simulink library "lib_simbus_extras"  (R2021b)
settings: Solver=ode45  StartTime=0.0  StopTime=10.0  RelTol=1e-3  EnableMultiTasking=on
undefined symbols (not defined in the file): BLOCKS, core, generic_inertance_pvs, measurement, SIMBUS, SIMBUS_BONDGRAPHS, SIMBUS_CORE, Timeseries
libraries: lib_select_power_variable x3

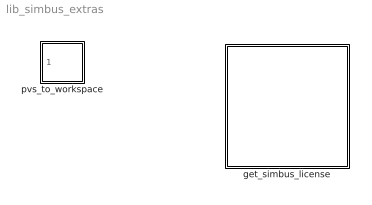
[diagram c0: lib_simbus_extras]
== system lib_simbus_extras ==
  get_simbus_license : Subsystem  mask(Get Simbus Products License){simbus_vendor=SIMBUS, simbus_toolbox=SIMBUS_CORE, simbus_component=BLOCKS, simbus_class=core.utils.get_simbus_license}
      mask prompts: simbus_vendor "Vendor:"; simbus_toolbox "Toolbox:"; simbus_component "Component:"; simbus_class "Class:"
      mask help: If you discover one or more missing library block in this model, then it is likely that you do not have a license to use Simbus products. Select the license that is most appropriate to your needs using one of the buttons below. If you are in receipt of this model from a third party (such as a project partner, contractor, or consultant) but do not need to modify it, then select the free Run-Time License. A Run-Time License is perpetual. If you wish to evaluate Simbus products for free, then select the free Trial License. A Trial License is a limited-duration license but is not limited in any wa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
  pvs_to_workspace : Subsystem  mask(Power Variables to Workspace){simbus_vendor=SIMBUS, simbus_toolbox=SIMBUS_BONDGRAPHS, simbus_component=BLOCKS, simbus_class=measurement.pvs_to_workspace, msk_var_name=generic_inertance_pvs, msk_max_datapoints=inf, msk_decimation=1, msk_save_format=Timeseries, msk_sample_time=-1, msk_apply_antialiasing=off}
      mask prompts: simbus_vendor "Vendor:"; simbus_toolbox "Toolbox:"; simbus_component "Component:"; simbus_class "Class:"; msk_var_name "Simulink:blkprm_prompts:ToWksVarName"; msk_max_datapoints "Simulink:blkprm_prompts:ToWksMaxDataPoints"; msk_decimation "Simulink:blkprm_prompts:AllBlksDecimation"; msk_save_format "Simulink:blkprm_prompts:ToWksSaveFormat"; msk_sample_time "Simulink:blkprm_prompts:AllBlksSampleTime"; msk_apply_antialiasing "Apply Antialiasing Filtering?"
      mask help: This block saves the generalized effort, generalized flow, and power of the connected bond to the MATLAB workspace. The user may optionally specify antialiasing filtering for these signals. The antialiasing filters are simple first-order filters with a cut-off frequency in Hertz set 1/(2*T), where T is a the sample period.
      mask init:
      | this_blk_bio = simbus_bio.factory(gcb);
      | apply_antialiasing = this_blk_bio{'apply_antialiasing'};
      | if apply_antialiasing
      | 
      |    Ts = this_blk_bio{'sample_time'};
      |    if Ts < 0
      |       errordlg('Failed to determine sample time.');
      |    elseif Ts > 0
      |       w_break = (pi/Ts);
      |       num_f = w_break;
      |       den_f = [1, w_break];
      |    else
      |       num_f = 1;
      |       den_f = 1;
      |    end % if Ts < 0
      | else % "apply_antialiasing" is false => pass-through
      | 
      |    num_f = 1;
      |    den_f = 1;
      | 
      | end % if apply_antialiasing

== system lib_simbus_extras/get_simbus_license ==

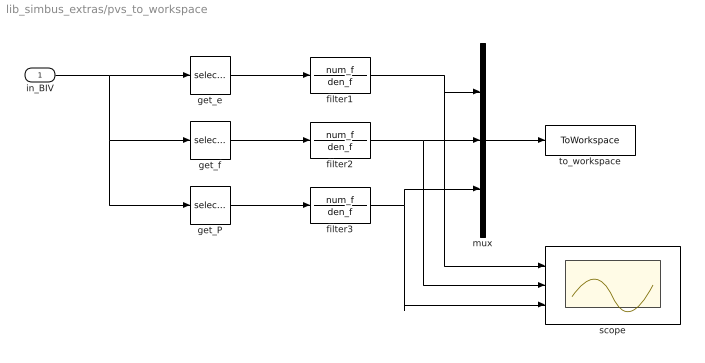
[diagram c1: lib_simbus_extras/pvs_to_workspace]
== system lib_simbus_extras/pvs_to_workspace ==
  in_BIV : Inport
  filter1 : TransferFcn  Numerator=num_f  Denominator=den_f
  filter2 : TransferFcn  Numerator=num_f  Denominator=den_f
  filter3 : TransferFcn  Numerator=num_f  Denominator=den_f
  get_P : lib_select_power_variable/select_power_variable  simbus_vendor=SIMBUS  simbus_toolbox=SIMBUS_BONDGRAPHS  simbus_component=BLOCKS  simbus_class=measurement.select_power_variable  msk_pv_idx=Power
  get_e : lib_select_power_variable/select_power_variable  simbus_vendor=SIMBUS  simbus_toolbox=SIMBUS_BONDGRAPHS  simbus_component=BLOCKS  simbus_class=measurement.select_power_variable  msk_pv_idx=Effort
  get_f : lib_select_power_variable/select_power_variable  simbus_vendor=SIMBUS  simbus_toolbox=SIMBUS_BONDGRAPHS  simbus_component=BLOCKS  simbus_class=measurement.select_power_variable  msk_pv_idx=Flow
  mux : Mux  Inputs=3
  scope : Scope  NumInputPorts=3
  to_workspace : ToWorkspace  VariableName=generic_inertance_pvs  SaveFormat=Timeseries  SampleTime=msk_sample_time
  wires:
  filter3/1 -> mux/3, scope/3
  get_P/1 -> filter3/1
  filter2/1 -> mux/2, scope/2
  get_f/1 -> filter2/1
  filter1/1 -> mux/1, scope/1
  get_e/1 -> filter1/1
  in_BIV/1 -> get_e/1, get_P/1, get_f/1
  mux/1 -> to_workspace/1
